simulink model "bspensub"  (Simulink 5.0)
settings: Solver=ode45  SolverMode=SingleTasking  StartTime=0.0  StopTime=10.0  FixedStep=0.01  RelTol=1e-3

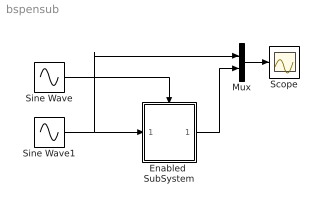
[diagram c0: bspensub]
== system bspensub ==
  Enabled  SubSystem : Subsystem
  Mux : Mux  Inputs=2
  Scope : Scope
  Sine Wave : Sin  SampleTime=0
  Sine Wave1 : Sin  SampleTime=0
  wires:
  Sine Wave1/1 -> Enabled  SubSystem/1(In1), Mux/1
  Sine Wave/1 -> Enabled  SubSystem/Enable
  Mux/1 -> Scope/1
  Enabled  SubSystem/1(Out1) -> Mux/2

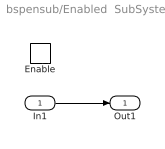
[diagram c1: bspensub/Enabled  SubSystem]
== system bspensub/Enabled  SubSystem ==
  In1 : Inport
  Enable : EnablePort
  Out1 : Outport
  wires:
  In1/1 -> Out1/1
